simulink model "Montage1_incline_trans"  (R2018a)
settings: Solver=VariableStepAuto  StartTime=0.0  StopTime=10.0  RelTol=1e-3
model workspace: external: MATLAB File (data not in the file)
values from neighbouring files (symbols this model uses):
  smiData = struct    [Montage1_DataFile.m]    (also in Montage2_DataFile.m)
undefined symbols (not defined in the file or in its folder): kg, m, mm, N, s, X, Y, Z
libraries: sm_lib x10, nesl_utility x1

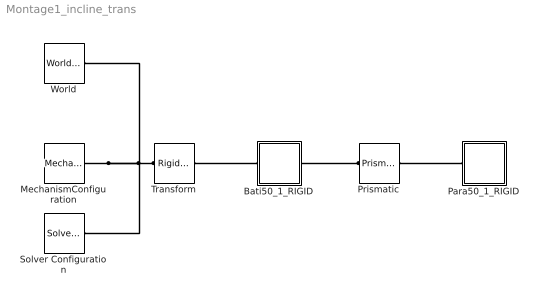
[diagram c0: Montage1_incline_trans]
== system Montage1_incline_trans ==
  Bati50_1_RIGID : Subsystem
  MechanismConfiguration : sm_lib/Utilities/Mechanism Configuration  UniformGravity=Constant  GravityVector=[0 -9.80665 0]  GravityUnits=m/s^2  LinearizationDelta=0.001
  Para50_1_RIGID : Subsystem
  Prismatic : sm_lib/Joints/Prismatic Joint  SenseConstraintForce=off  SenseConstraintForceX=off  SenseConstraintForceY=off  SenseConstraintForceZ=off  SenseConstraintTorque=off  SenseConstraintTorqueX=off  SenseConstraintTorqueY=off  SenseConstraintTorqueZ=off  SenseTotalForce=off  SenseTotalForceX=off  SenseTotalForceY=off  SenseTotalForceZ=off  SenseTotalTorque=off  SenseTotalTorqueX=off  SenseTotalTorqueY=off  SenseTotalTorqueZ=off  CompositeWrenchDir=FollowerOnBase  CompositeWrenchFrame=BaseFrame  EquilibriumPosition=0  EquilibriumPositionUnits=m  SpringStiffness=0  SpringStiffnessUnits=N/m  DampingCoefficient=0  DampingCoefficientUnits=N/(m/s)  TorqueActuationMode=NoTorque  MotionActuationMode=ComputedMotion  SensePosition=off  SenseVelocity=off  SenseAcceleration=off  SenseTorqueForce=off  PositionTargetSpecify=on  PositionTargetPriority=Low  PositionTargetValue=smiData.PrismaticJoint(1).Pz.Pos  PositionTargetValueUnits=m  VelocityTargetSpecify=off  VelocityTargetPriority=High  VelocityTargetValue=0  VelocityTargetValueUnits=m/s
  Solver Configuration : nesl_utility/Solver Configuration  PhysicalDomain=network_engine_domain  SubClassName=solver  LeftPortType=input  RightPortType=generic  Tones=[]  Harmonics=[]  SimulateNoise=off  Profile=off  UseLocalSampling=off  EnableSwitchedLinearOptims=on  FrequencyDomain=off  UseCCode=off  RelTol=0.001  AbsTol=1e-06  MinStep=1e-09  ToWorkspace=off  RevertToSquareIcSolve=off  NumHomotopyIterations=100  PhasorMode=off  PhasorModeNumHarmonics=1  DoDC=off  ResidualTolerance=1e-09  UseLocalSolver=off  LocalSolverChoice=NE_BACKWARD_EULER_ADVANCER  LocalSolverSampleTime=0.001  DoFixedCost=off  MaxNonlinIter=3  MaxModeIter=2  LinearAlgebra=Sparse  EquationFormulation=NE_TIME_EF  DelaysMemoryBudget=1024  AutomaticFiltering=on  FilteringTimeConstant=0.001
  Transform : sm_lib/Frames and Transforms/Rigid Transform  TranslationMethod=Cartesian  TranslationStandardOffset=0  TranslationLengthUnit=mm  TranslationStandardAxis=+Z  TranslationCartesianOffset=smiData.RigidTransform(3).translation  TranslationROffset=0  TranslationROffsetUnits=m  TranslationZOffset=0  TranslationZOffsetUnits=m  TranslationThetaOffset=0  TranslationThetaOffsetUnits=deg  RotationMethod=StandardAxis  RotationAngleUnits=deg  RotationStandardAxis=+X  RotationAngle=30  RotationArbitraryAxis=smiData.RigidTransform(3).axis  FollAlignAxisA=+X  BaseAlignAxisA=+Y  FollAlignAxisB=+Y  BaseAlignAxisB=+Z  RotationSequenceAxes=FollowerAxes  RotationSequence=XYX  RotationSequenceAngles=[0 0 0]  RotationSequenceAnglesUnits=deg  RotationMatrix=[1 0 0; 0 1 0; 0 0 1]
  World : sm_lib/Frames and Transforms/World Frame
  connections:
  Transform/LConn1 -- MechanismConfiguration/RConn1 -- Solver Configuration/RConn1 -- World/RConn1
  Bati50_1_RIGID/RConn1 -- Prismatic/LConn1
  Para50_1_RIGID/LConn1 -- Prismatic/RConn1
  Bati50_1_RIGID/LConn1 -- Transform/RConn1

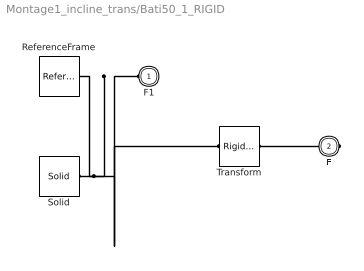
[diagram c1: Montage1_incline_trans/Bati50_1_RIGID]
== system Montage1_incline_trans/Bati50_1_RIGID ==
  ReferenceFrame : sm_lib/Frames and Transforms/Reference Frame
  Solid : sm_lib/Body Elements/Solid  InertiaType=Custom  Mass=smiData.Solid(2).mass  MassUnits=kg  CenterOfMass=smiData.Solid(2).CoM  CenterOfMassUnits=mm  MomentsOfInertia=smiData.Solid(2).MoI  MomentsOfInertiaUnits=kg*mm^2  ProductsOfInertia=smiData.Solid(2).PoI  ProductsOfInertiaUnits=kg*mm^2  DensityBased=on  Density=1000  DensityUnits=kg/m^3  DoExposeReferenceFrame=on  SerializedFrames=<Frames/>  GraphicType=FromGeometry  MarkerShape=Sphere  MarkerSize=10  GraphicVisPropType=SimpleVisualProperties  GraphicDiffuseColor=smiData.Solid(2).color  GraphicSpecularColor=[0.5 0.5 0.5 1.0]  GraphicAmbientColor=[0.15 0.15 0.15 1.0]  GraphicEmissiveColor=[0.0 0.0 0.0 1.0]  GraphicShininess=75  GraphicOpacity=smiData.Solid(2).opacity  GeometryShape=FromFile  RectangleSize=[1 1]  RectangleSizeUnits=m  BrickDimensions=[1 1 1]  BrickDimensionUnits=m  CylinderRadius=1  CylinderRadiusUnits=m  CylinderLength=1  CylinderLengthUnits=m  SphereRadius=1  SphereRadiusUnits=m  EllipsoidRadii=[1 1 1]  EllipsoidRadiiUnits=m  ExtrusionCrossSection=[1 1; -1 1; -1 -1; 1 -1]  ExtrusionCrossSectionUnits=m  ExtrusionLength=1  ExtrusionLengthUnits=m  PolygonNumSides=3  PolygonOuterRadius=1  PolygonOuterRadiusUnits=m  ExtGeomFileType=STEP  ExtGeomFileName=Bati50_Défaut_sldprt.STEP  ExtGeomFileUnits=m  RevolutionCrossSection=[1 1; 1 -1; 2 -1; 2 1]  RevolutionCrossSectionUnits=m  RevolutionExtent=Full  RevolutionAngle=180  RevolutionAngleUnits=deg
  Transform : sm_lib/Frames and Transforms/Rigid Transform  TranslationMethod=Cartesian  TranslationStandardOffset=0  TranslationLengthUnit=mm  TranslationStandardAxis=+Z  TranslationCartesianOffset=smiData.RigidTransform(1).translation  TranslationROffset=0  TranslationROffsetUnits=m  TranslationZOffset=0  TranslationZOffsetUnits=m  TranslationThetaOffset=0  TranslationThetaOffsetUnits=deg  RotationMethod=ArbitraryAxis  RotationAngleUnits=rad  RotationStandardAxis=+Z  RotationAngle=smiData.RigidTransform(1).angle  RotationArbitraryAxis=smiData.RigidTransform(1).axis  FollAlignAxisA=+X  BaseAlignAxisA=+Y  FollAlignAxisB=+Y  BaseAlignAxisB=+Z  RotationSequenceAxes=FollowerAxes  RotationSequence=XYX  RotationSequenceAngles=[0 0 0]  RotationSequenceAnglesUnits=deg  RotationMatrix=[1 0 0; 0 1 0; 0 0 1]
  F1 : PMIOPort  Side=Left
  F : PMIOPort  Port=2  Side=Right
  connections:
  Solid/RConn1 -- ReferenceFrame/RConn1 -- Transform/LConn1 -- F1/RConn1
  Transform/RConn1 -- F/RConn1

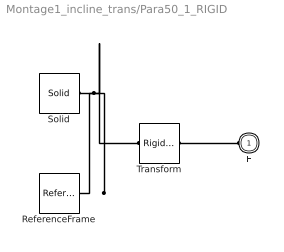
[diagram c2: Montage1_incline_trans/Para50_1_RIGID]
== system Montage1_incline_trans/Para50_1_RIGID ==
  ReferenceFrame : sm_lib/Frames and Transforms/Reference Frame
  Solid : sm_lib/Body Elements/Solid  InertiaType=Custom  Mass=smiData.Solid(1).mass  MassUnits=kg  CenterOfMass=smiData.Solid(1).CoM  CenterOfMassUnits=mm  MomentsOfInertia=smiData.Solid(1).MoI  MomentsOfInertiaUnits=kg*mm^2  ProductsOfInertia=smiData.Solid(1).PoI  ProductsOfInertiaUnits=kg*mm^2  DensityBased=on  Density=1000  DensityUnits=kg/m^3  DoExposeReferenceFrame=on  SerializedFrames=<Frames/>  GraphicType=FromGeometry  MarkerShape=Sphere  MarkerSize=10  GraphicVisPropType=SimpleVisualProperties  GraphicDiffuseColor=[1.0 0.0 0.2]  GraphicSpecularColor=[0.5 0.5 0.5 1.0]  GraphicAmbientColor=[0.15 0.15 0.15 1.0]  GraphicEmissiveColor=[0.0 0.0 0.0 1.0]  GraphicShininess=75  GraphicOpacity=smiData.Solid(1).opacity  GeometryShape=FromFile  RectangleSize=[1 1]  RectangleSizeUnits=m  BrickDimensions=[1 1 1]  BrickDimensionUnits=m  CylinderRadius=1  CylinderRadiusUnits=m  CylinderLength=1  CylinderLengthUnits=m  SphereRadius=1  SphereRadiusUnits=m  EllipsoidRadii=[1 1 1]  EllipsoidRadiiUnits=m  ExtrusionCrossSection=[1 1; -1 1; -1 -1; 1 -1]  ExtrusionCrossSectionUnits=m  ExtrusionLength=1  ExtrusionLengthUnits=m  PolygonNumSides=3  PolygonOuterRadius=1  PolygonOuterRadiusUnits=m  ExtGeomFileType=STEP  ExtGeomFileName=Para50_Défaut_sldprt.STEP  ExtGeomFileUnits=m  RevolutionCrossSection=[1 1; 1 -1; 2 -1; 2 1]  RevolutionCrossSectionUnits=m  RevolutionExtent=Full  RevolutionAngle=180  RevolutionAngleUnits=deg
  Transform : sm_lib/Frames and Transforms/Rigid Transform  TranslationMethod=Cartesian  TranslationStandardOffset=0  TranslationLengthUnit=mm  TranslationStandardAxis=+Z  TranslationCartesianOffset=smiData.RigidTransform(2).translation  TranslationROffset=0  TranslationROffsetUnits=m  TranslationZOffset=0  TranslationZOffsetUnits=m  TranslationThetaOffset=0  TranslationThetaOffsetUnits=deg  RotationMethod=ArbitraryAxis  RotationAngleUnits=rad  RotationStandardAxis=+Z  RotationAngle=smiData.RigidTransform(2).angle  RotationArbitraryAxis=smiData.RigidTransform(2).axis  FollAlignAxisA=+X  BaseAlignAxisA=+Y  FollAlignAxisB=+Y  BaseAlignAxisB=+Z  RotationSequenceAxes=FollowerAxes  RotationSequence=XYX  RotationSequenceAngles=[0 0 0]  RotationSequenceAnglesUnits=deg  RotationMatrix=[1 0 0; 0 1 0; 0 0 1]
  F : PMIOPort  Side=Left
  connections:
  Solid/RConn1 -- ReferenceFrame/RConn1 -- Transform/LConn1
  Transform/RConn1 -- F/RConn1
